|Texas Instruments Incorporated
|tmux1309, 2 Data Lane 4_1x2 5V Precision mux
[IBIS Ver]   4.1
[File name]   tmux1309.ibs
[Date]   07/12/22
[File Rev]   1.0
[Source]
| Texas Instruments Incorporated.
| ASC-INT-MPD
| 12500 TI Blvd
| Dallas, TX - 75243
[Notes]   Revision History:
| Rev 1.0: 07/12/22
| - Initial version of the model
| - Model generated from simulations in SPECTRE
| - C_comp although listed in numerical order of value are
|   obtained from varying PVT conditions. For PVT conditions for
|   each specific value refer the buffer description under
|   respective [Model]. IBIS model user is responsible for using
|   appropriate C_comp to simulate for Signal Integrity.
[Disclaimer]
| This model is designed as an aid for customers of Texas Instruments.
| TI and its licensors and suppliers make no warranties, either expressed
| or implied, with respect to this  model, including the warranties of
| merchantability or fitness for a particular purpose. The model is
| provided solely on an "as is" basis. The entire risk as to its quality
| and performance is with the customer.
| This model is subject to change without notice. Texas Instruments
| Incorporated is not responsible for updating this model.
[Copyright]
(C) Copyright 2022 Texas Instruments Incorporated.All rights reserved.
|  Component TMUX1309PW 16-pin - PW package
|  Part # TMUX1309PW
[Component]   TMUX1309PW
[Manufacturer]  TI
[Package]
|   typ   min   max
R_pkg   0.0668   NA   NA
L_pkg   2.1992nH   NA   NA
C_pkg   0.2884pF   NA   NA
[Pin]   signal_name   model_name
   1   S0B   sterm
   2   S2B   sterm
   3   DB   dterm
   4   S3B   sterm
   5   S1B   sterm
   6   ENZ_5P5_PAD   inbuf
   7   NC   nc
   8   GND   gnd
   9   A1   inbuf
   10   A0   inbuf
   11   S3A   sterm
   12   S0A   sterm
   13   DA   dterm
   14   S1A   sterm
   15   S2A   sterm
   16   VDD   power
[Series Switch Groups]
On 1 /
On 2 /
On 3 /
On 4 /
Off 1 2 3 4 /
[Series Pin Mapping]  pin_2 model_name function_table_group
   1   3   switch_1.8   1
  12  13   switch_1.8   1
   5   3   switch_1.8   2
  14  13   switch_1.8   2
   2   3   switch_1.8   3
  15  13   switch_1.8   3
   4   3   switch_1.8   4
  11  13   switch_1.8   4
|   1   3   switch_3.3   1
|  12  13   switch_3.3   1
|   5   3   switch_3.3   2
|  14  13   switch_3.3   2
|   2   3   switch_3.3   3
|  15  13   switch_3.3   3
|   4   3   switch_3.3   4
|  11  13   switch_3.3   4
|   1   3   switch_2.5   1
|  12  13   switch_2.5   1
|   5   3   switch_2.5   2
|  14  13   switch_2.5   2
|   2   3   switch_2.5   3
|  15  13   switch_2.5   3
|   4   3   switch_2.5   4
|  11  13   switch_2.5   4
|   1   3   switch_5   1
|  12  13   switch_5   1
|   5   3   switch_5   2
|  14  13   switch_5   2
|   2   3   switch_5   3
|  15  13   switch_5   3
|   4   3   switch_5   4
|  11  13   switch_5   4
|  Component TMUX1309DYY 16-pin - DYY package
|  Part # TMUX1309DYY
[Component]   TMUX1309DYY
[Manufacturer]  TI
[Package]
|   typ   min   max
R_pkg   0.0668   NA   NA
L_pkg   2.1992nH   NA   NA
C_pkg   0.2884pF   NA   NA
[Pin]   signal_name   model_name
   1   S0B   sterm
   2   S2B   sterm
   3   DB   dterm
   4   S3B   sterm
   5   S1B   sterm
   6   ENZ_5P5_PAD   inbuf
   7   NC   nc
   8   GND   gnd
   9   A1   inbuf
   10   A0   inbuf
   11   S3A   sterm
   12   S0A   sterm
   13   DA   dterm
   14   S1A   sterm
   15   S2A   sterm
   16   VDD   power
[Series Switch Groups]
On 1 /
On 2 /
On 3 /
On 4 /
Off 1 2 3 4 /
[Series Pin Mapping]  pin_2 model_name function_table_group
   1   3   switch_1.8   1
  12  13   switch_1.8   1
   5   3   switch_1.8   2
  14  13   switch_1.8   2
   2   3   switch_1.8   3
  15  13   switch_1.8   3
   4   3   switch_1.8   4
  11  13   switch_1.8   4
|   1   3   switch_3.3   1
|  12  13   switch_3.3   1
|   5   3   switch_3.3   2
|  14  13   switch_3.3   2
|   2   3   switch_3.3   3
|  15  13   switch_3.3   3
|   4   3   switch_3.3   4
|  11  13   switch_3.3   4
|   1   3   switch_2.5   1
|  12  13   switch_2.5   1
|   5   3   switch_2.5   2
|  14  13   switch_2.5   2
|   2   3   switch_2.5   3
|  15  13   switch_2.5   3
|   4   3   switch_2.5   4
|  11  13   switch_2.5   4
|   1   3   switch_5   1
|  12  13   switch_5   1
|   5   3   switch_5   2
|  14  13   switch_5   2
|   2   3   switch_5   3
|  15  13   switch_5   3
|   4   3   switch_5   4
|  11  13   switch_5   4
|  Component TMUX1309BQB 16-pin - BQB package
|  Part # TMUX1309BQB
[Component]   TMUX1309BQB
[Manufacturer]  TI
[Package]
|   typ   min   max
R_pkg   0.0668   NA   NA
L_pkg   2.1992nH   NA   NA
C_pkg   0.2884pF   NA   NA
[Pin]   signal_name   model_name
   1   S0B   sterm
   2   S2B   sterm
   3   DB   dterm
   4   S3B   sterm
   5   S1B   sterm
   6   ENZ_5P5_PAD   inbuf
   7   NC   nc
   8   GND   gnd
   9   A1   inbuf
   10   A0   inbuf
   11   S3A   sterm
   12   S0A   sterm
   13   DA   dterm
   14   S1A   sterm
   15   S2A   sterm
   16   VDD   power
[Series Switch Groups]
On 1 /
On 2 /
On 3 /
On 4 /
Off 1 2 3 4 /
[Series Pin Mapping]  pin_2 model_name function_table_group
   1   3   switch_1.8   1
  12  13   switch_1.8   1
   5   3   switch_1.8   2
  14  13   switch_1.8   2
   2   3   switch_1.8   3
  15  13   switch_1.8   3
   4   3   switch_1.8   4
  11  13   switch_1.8   4
|   1   3   switch_3.3   1
|  12  13   switch_3.3   1
|   5   3   switch_3.3   2
|  14  13   switch_3.3   2
|   2   3   switch_3.3   3
|  15  13   switch_3.3   3
|   4   3   switch_3.3   4
|  11  13   switch_3.3   4
|   1   3   switch_2.5   1
|  12  13   switch_2.5   1
|   5   3   switch_2.5   2
|  14  13   switch_2.5   2
|   2   3   switch_2.5   3
|  15  13   switch_2.5   3
|   4   3   switch_2.5   4
|  11  13   switch_2.5   4
|   1   3   switch_5   1
|  12  13   switch_5   1
|   5   3   switch_5   2
|  14  13   switch_5   2
|   2   3   switch_5   3
|  15  13   switch_5   3
|   4   3   switch_5   4
|  11  13   switch_5   4
[Model Selector] dterm
dterm_1.8 Use for operation at 1V
dterm_3.3 Use for operation at 3V
dterm_2.5 Use for operation at 2V
dterm_5 Use for operation at 5V
[Model Selector] sterm
sterm_1.8 Use for operation at 1V
sterm_3.3 Use for operation at 3V
sterm_2.5 Use for operation at 2V
sterm_5 Use for operation at 5V
[Model Selector] inbuf
inbuf_1.8 Use for operation at 1V
inbuf_3.3 Use for operation at 3V
inbuf_2.5 Use for operation at 2V
inbuf_5 Use for operation at 5V
| switch_1.8
[Model]   switch_1.8
Model_type   Series_switch
|   typ   min   max
C_comp   1.008417e-12   NA   NA
[Voltage Range]   1.8   NA   NA
[Power Clamp Reference]   1.8   NA   NA
[Temperature Range]   27   NA   NA
[On]
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[Off]
|   typ   min   max
[R Series]   10G   NA   NA
| switch_3.3
[Model]   switch_3.3
Model_type   Series_switch
|   typ   min   max
C_comp   1.008417e-12   NA   NA
[Voltage Range]   3.3   NA   NA
[Power Clamp Reference]   3.3   NA   NA
[Temperature Range]   27   NA   NA
[On]
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[Off]
|   typ   min   max
[R Series]   10G   NA   NA
| switch_2.5
[Model]   switch_2.5
Model_type   Series_switch
|   typ   min   max
C_comp   1.008417e-12   NA   NA
[Voltage Range]   2.5   NA   NA
[Power Clamp Reference]   2.5   NA   NA
[Temperature Range]   27   NA   NA
[On]
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[Off]
|   typ   min   max
[R Series]   10G   NA   NA
| switch_5
[Model]   switch_5
Model_type   Series_switch
|   typ   min   max
C_comp   1.598234e-12   NA   NA
[Voltage Range]   5   NA   NA
[Power Clamp Reference]   5   NA   NA
[Temperature Range]   27   NA   NA
[On]
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[Off]
|   typ   min   max
[R Series]   10G   NA   NA
| Models and submodels in the file (16): dterm_1.8 (Terminator), dterm_3.3 (Terminator), dterm_2.5 (Terminator), dterm_5 (Terminator), switch_1.8 (Series_switch), switch_3.3 (Series_switch), switch_2.5 (Series_switch), switch_5 (Series_switch), sterm_1.8 (Terminator), sterm_3.3 (Terminator), sterm_2.5 (Terminator), sterm_5 (Terminator), inbuf_1.8 (Input), inbuf_3.3 (Input), inbuf_2.5 (Input), inbuf_5 (Input)
